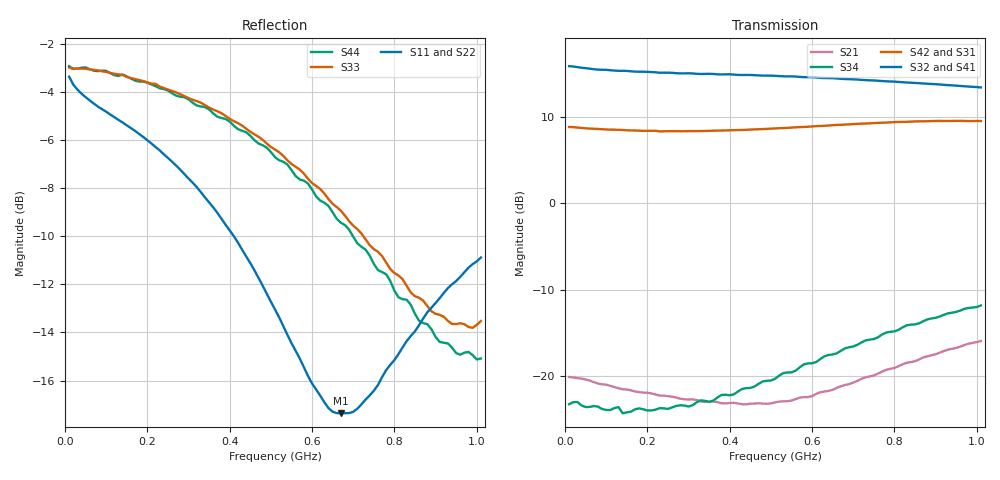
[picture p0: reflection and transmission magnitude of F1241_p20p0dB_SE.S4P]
! Integrated Device Technology
! Corporate Headquarters
! 6024 Silver Creek Valley Road
! San Jose, CA 95138  USA
! Phone:  1-408-284-8200
! Toll Free:  1-800-223-1366
! Webpage:  http://www.idt.com/
! Timing and RF Division
! 515 Groton Road, Suite 102
! Westford, MA 01886-6024
! Device:  F1241
! Description: Dual Intermediate Frequency Digital Variable Gain Amplifier
! Frequency:  10.0 -  500.00 MHz
! Package:  5x5 mm QFN Plastic Package: 32 pin
! Ports:  8 RF, 20 DC
!  Pin  1  = GA3  Pin 17  = RF OUT_B+
!  Pin  2  = GA4  Pin 18  = RF OUT_B-
!  Pin  3  = GA5  Pin 19  = STBY_B
!  Pin  4  = ISET_A  Pin 20  = Ground
!  Pin  5  = ISET_B  Pin 21  = Ground
!  Pin  6  = GB5  Pin 22  = STB_A
!  Pin  7  = GB4  Pin 23  = RF OUT_A-  = Port 4
!  Pin  8  = GB3  Pin 24  = RF OUT_A+  = Port 3
!  Pin  9  = GB2  Pin 25  = NO CONNECT
!  Pin 10  = GB1  Pin 26  = NO CONNECT
!  Pin 11  = RF IN_B+  Pin 27  = VCC
!  Pin 12  = RF IN_B-  Pin 28  = Ground
!  Pin 13  = Ground  Pin 29  = RF IN_A-  = Port 2
!  Pin 14  = VCC  Pin 30  = RF IN_A+  = Port 1
!  Pin 15  = NO CONNECT  Pin 31  = GA1
!  Pin 16  = NO CONNECT  Pin 32  = GA2
! State:  0
! Gain State:  20.0 dB
! Voltages:  Vcc = +5.00 Volts  Icc approximately 160.0 mA or 80 mA per channel.
! Data:  The device was measured on a custom evaluation board which has
!  individual transmission lines to the RF pins.  Data was collected
!  using a calibrated network analyzer.  The evaluation board was
!  de-embedded using a port reference technique.
!  The reference plane is the edge of the package pin.
!  Only Channel A was measured.
!  This data is in single-ended operation.  If your needs are balanced
!  or differential S-parameters then this file needs to be used a
!  linear simulator.
! Misc:  Lot Code  160028MY
!  Action Tracker AT004
! Date Measured:  2014-08-14
! Date:  2014-08-28  MJV
! Note:
!  Integrated Device Technology supplies this data as a sample of measured
!  data at the package pin for this product.  Your particular data for this
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# Hz S dB R 50
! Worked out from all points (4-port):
!   101 points, 10 MHz to 1.01 GHz, reference 50 ohm
!   strongest paths, dB at 10 MHz, 260 MHz, 510 MHz, 760 MHz, 1.01 GHz:
!     S32: 15.9, 15.1, 14.8, 14.2, 13.4
!     S41: 15.9, 15.0, 14.6, 13.9, 13.1
!     S42: 8.8, 8.4, 8.7, 9.3, 9.5
!     S31: 8.8, 8.2, 8.4, 9.0, 9.3
!     S34: -23.2, -23.6, -20.3, -15.5, -11.8
!     S21: -20.1, -22.4, -23.0, -19.7, -15.9
!   lowest |S11| = -17.4 dB at 670 MHz (marker M1), VSWR 1.31, Z = 39.7 - j6.47 ohm
!   |S11| at or under -10 dB: 410 MHz to end of sweep
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1e7  -3.38 -8.7  -20.06 6.9  -50.19 39.2  -26.32 4.4
     -20.10 6.8  -3.38 -8.6  -26.36 4.1  -50.37 39.9
     8.83 5.3  15.88 -173.8  -3.00 -5.0  -23.25 14.4
     15.89 -173.8  8.84 5.4  -23.18 13.4  -2.94 -5.2
3e7  -3.91 -9.9  -20.20 -5.9  -47.17 50.6  -26.42 -1.3
     -20.23 -5.7  -3.91 -9.7  -26.47 -0.8  -47.37 50.1
     8.75 -2.1  15.77 176.9  -3.03 -3.7  -22.99 -5.9
     15.79 176.7  8.78 -2.1  -23.14 -4.4  -3.04 -3.5
6e7  -4.36 -13.5  -20.62 -15.3  -42.78 62.7  -26.72 -2.1
     -20.52 -15.6  -4.39 -12.9  -26.71 -2.4  -42.90 63.6
     8.67 -7.1  15.59 171.2  -3.07 -5.7  -23.56 -14.7
     15.58 170.9  8.66 -6.8  -23.49 -14.4  -3.06 -5.9
2.8e8  -7.24 -40.5  -22.54 -58.9  -30.51 54.2  -26.29 -2.5
       -22.60 -62.3  -7.15 -38.6  -26.28 -2.4  -30.48 54.1
       8.17 -29.7  15.05 143.4  -4.11 -21.8  -23.37 -72.8
       14.98 142.5  8.35 -29.4  -25.25 -71.3  -4.21 -20.4
4.9e8  -12.39 -75.4  -23.33 -116.5  -26.06 34.0  -24.70 -10.2
       -23.19 -121.6  -12.27 -72.3  -24.55 -10.2  -25.93 33.0
       8.30 -48.7  14.79 117.9  -6.16 -38.5  -20.54 -131.1
       14.63 116.7  8.62 -49.5  -23.46 -137.0  -6.32 -35.8
6.7e8  -17.36 -143.8  -21.92 -175.8  -24.01 15.1  -23.76 -24.1
       -21.17 179.8  -17.73 -138.9  -23.48 -24.2  -23.83 13.6
       8.74 -67.2  14.42 95.5  -8.94 -56.4  -17.07 -175.4
       14.20 94.5  9.09 -69.3  -19.00 168.3  -9.44 -50.4
1.01e9  -10.89 133.8  -16.21 107.2  -22.36 -16.3  -24.32 -55.2
        -15.93 103.9  -10.98 136.3  -23.77 -54.6  -22.11 -19.2
        9.27 -111.8  13.42 53.1  -13.53 -121.1  -11.82 114.4
        13.12 52.4  9.53 -115.3  -12.58 100.2  -15.08 -113.9
